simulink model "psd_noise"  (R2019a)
settings: Solver=ode45  StartTime=0.0  StopTime=10.0  RelTol=1e-3  EnableMultiTasking=on
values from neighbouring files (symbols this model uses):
  ampl1 = 10    [psd_noise_4.m]
  ampl2 = 5    [psd_noise_4.m]
  fsig1 = 100.5    [psd_noise_4.m]
  fsig2 = 150.3    [psd_noise_4.m]
  N = 1024    [psd_noise_4.m]    (also in leakage_1.m = 20; fenster_funkt_2.m; fenstereffekte_3.m)
  noise = 2    [psd_noise_4.m]
  phi1 = pi/3    (= 1.0471975512)    [psd_noise_4.m]
  phi2 = pi/5    (= 0.628318530718)    [psd_noise_4.m]
  pw = sum(hanning(N).^2)/N    [psd_noise_4.m]    (also in fenstereffekte_3.m)
  Ts = 1/fs    (= 0.0009765625)    [psd_noise_4.m]    (also in leakage_1.m = 0.05; fenstereffekte_3.m)
libraries: dspspect3 x2, dspstat3 x2, dspsigops x2

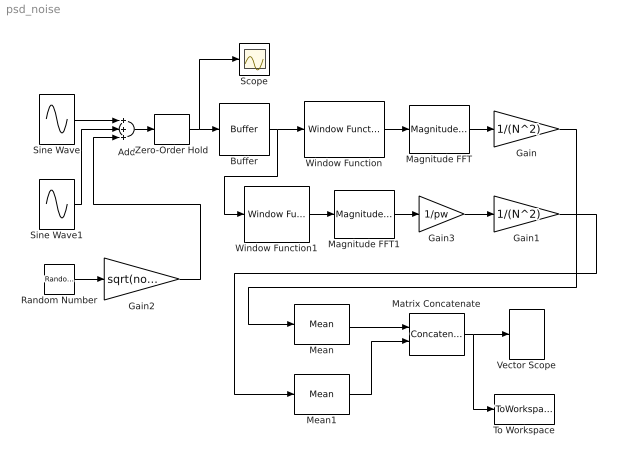
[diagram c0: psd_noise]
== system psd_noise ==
  Add : Sum  Inputs=+++
  Buffer : Buffer  N=N
  Gain : Gain  Gain=1/(N^2)
  Gain1 : Gain  Gain=1/(N^2)
  Gain2 : Gain  Gain=sqrt(noise)
  Gain3 : Gain  Gain=1/pw
  Magnitude FFT : dspspect3/Magnitude FFT  mag_or_magsq=Magnitude squared  FFTImplementation=Auto  fftLenInherit=on  fftsize=256  WrapInput=on
  Magnitude FFT1 : dspspect3/Magnitude FFT  mag_or_magsq=Magnitude squared  FFTImplementation=Auto  fftLenInherit=on  fftsize=256  WrapInput=on
  Matrix Concatenate : Concatenate  Mode=Multidimensional array  ConcatenateDimension=2
  Mean : dspstat3/Mean  run=on  reset_popup=None  directionMode=Each column  dimension=1  roiEnable=off  roiType=Rectangles  roiPortion=Entire ROI  roiOutput=Individual statistics for each ROI  roiFlag=off  roundingMode=Floor  overflowMode=off  outputDataTypeStr=Inherit: Same as accumulator  outputMin=[]  outputMax=[]  outputLastDataTypeStr=Inherit: Same as accumulator
  Mean1 : dspstat3/Mean  run=on  reset_popup=None  directionMode=Each column  dimension=1  roiEnable=off  roiType=Rectangles  roiPortion=Entire ROI  roiOutput=Individual statistics for each ROI  roiFlag=off  roundingMode=Floor  overflowMode=off  outputDataTypeStr=Inherit: Same as accumulator  outputMin=[]  outputMax=[]  outputLastDataTypeStr=Inherit: Same as accumulator
  Random Number : RandomNumber  SampleTime=0
  Scope : Scope
  Sine Wave : Sin  Amplitude=ampl1  Frequency=2*pi*fsig1  Phase=phi1  SampleTime=0
  Sine Wave1 : Sin  Amplitude=ampl2  Frequency=2*pi*fsig2  Phase=phi2  SampleTime=0
  To Workspace : ToWorkspace  VariableName=Y  SampleTime=-1
  Vector Scope : SpectrumAnalyzer
  Window Function : dspsigops/Window Function  winmode=Apply window to input  wintype=Boxcar  sampmode=Continuous  samptime=1  N=64  Rs=50  beta=10  winsamp=Symmetric  UserWindow=fenster  OptParams=on  UserParams={'symmetric'}  dataType=double  isSigned=on  wordLen=16  udDataType=sfix(16)  fracBitsMode=Best precision  numFracBits=15  roundingMode=Floor  overflowMode=off  numSidelobes=4  sidelobeLevel=-30
  Window Function1 : dspsigops/Window Function  winmode=Apply window to input  wintype=Hanning  sampmode=Continuous  samptime=1  N=64  Rs=50  beta=10  winsamp=Symmetric  UserWindow=fenster  OptParams=on  UserParams={'symmetric'}  dataType=double  isSigned=on  wordLen=16  udDataType=sfix(16)  fracBitsMode=Best precision  numFracBits=15  roundingMode=Floor  overflowMode=off  numSidelobes=4  sidelobeLevel=-30
  Zero-Order Hold : ZeroOrderHold  SampleTime=Ts
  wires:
  Zero-Order Hold/1 -> Scope/1, Buffer/1
  Buffer/1 -> Window Function1/1, Window Function/1
  Magnitude FFT/1 -> Gain/1
  Window Function/1 -> Magnitude FFT/1
  Magnitude FFT1/1 -> Gain3/1
  Gain1/1 -> Mean1/1
  Gain/1 -> Mean/1
  Matrix Concatenate/1 -> To Workspace/1, Vector Scope/1
  Add/1 -> Zero-Order Hold/1
  Sine Wave/1 -> Add/1
  Sine Wave1/1 -> Add/2
  Random Number/1 -> Gain2/1
  Gain2/1 -> Add/3
  Mean/1 -> Matrix Concatenate/1
  Mean1/1 -> Matrix Concatenate/2
  Window Function1/1 -> Magnitude FFT1/1
  Gain3/1 -> Gain1/1
